DATA_BLOCK "Segnal Avvisi Allarmi OP"
TITLE =Segnalazioni Avvisi Allarmi OP17
AUTHOR : MassimoZ
FAMILY : NovaSrl
VERSION : 0.1


  STRUCT
   Avviso : BOOL ;	//Manca Marcia Generale
   Avviso1 : BOOL ;	//Barriere di sicurezza aperte
   Avviso2 : BOOL ;	//Protezioni anteriori aperte
   Avviso3 : BOOL ;	//Blocco cancello attivo
   Avviso4 : BOOL ;	//spare
   Avviso5 : BOOL ;	//spare
   Avviso6 : BOOL ;	//spare
   Avviso7 : BOOL ;	//spare
   Avviso8 : BOOL ;	//spare
   Avviso9 : BOOL ;	//spare
   Avviso10 : BOOL ;	//spare
   Avviso11 : BOOL ;	//spare
   Avviso12 : BOOL ;	//spare
   Avviso13 : BOOL ;	//spare
   Avviso14 : BOOL ;	//spare
   Avviso15 : BOOL ;	//spare
   Avviso16 : BOOL ;	//Inserito Arresto a Fine Ciclo
   Avviso17 : BOOL ;	//Eseguire Ref Point Assi
   Avviso18 : BOOL ;	//Testa Fuori Posizione Base per il Ciclo Aut
   Avviso19 : BOOL ;	//Testa Fuori Posizione Base per il Ciclo S/Aut
   Avviso20 : BOOL ;	//spare
   Avviso21 : BOOL ;	//spare
   Avviso22 : BOOL ;	//spare
   Avviso23 : BOOL ;	//Controllo corti escluso Escluso
   Avviso24 : BOOL ;	//Macchin in ingombro
   Avviso25 : BOOL ;	//Batteria Tampone Plc Scarica
   Avviso26 : BOOL ;
   Avviso27 : BOOL ;
   Avviso28 : BOOL ;
   Avviso29 : BOOL ;
   Avviso30 : BOOL ;
   Avviso31 : BOOL ;
   Avviso32 : BOOL ;
   Avviso33 : BOOL ;
   Avviso34 : BOOL ;
   Avviso35 : BOOL ;
   Avviso36 : BOOL ;
   Avviso37 : BOOL ;
   Avviso38 : BOOL ;
   Avviso39 : BOOL ;
   Avviso40 : BOOL ;
   Avviso41 : BOOL ;
   Avviso42 : BOOL ;
   Avviso43 : BOOL ;
   Avviso44 : BOOL ;
   Avviso45 : BOOL ;
   Avviso46 : BOOL ;
   Avviso47 : BOOL ;
   Avviso48 : BOOL ;
   Avviso49 : BOOL ;
   Avviso50 : BOOL ;
   Avviso51 : BOOL ;
   Avviso52 : BOOL ;
   Avviso53 : BOOL ;
   Avviso54 : BOOL ;
   Avviso55 : BOOL ;
   Avviso56 : BOOL ;
   Avviso57 : BOOL ;
   Avviso58 : BOOL ;
   Avviso59 : BOOL ;
   Avviso60 : BOOL ;
   Avviso61 : BOOL ;
   Avviso62 : BOOL ;
   Avviso63 : BOOL ;
   Allarme : BOOL ;	//Alimentazione Ausiliari 110Vac
   Allarme1 : BOOL ;	//Scatto termico IM1
   Allarme2 : BOOL ;	//Scatto termico IM2
   Allarme3 : BOOL ;	//Scatto termico IM3
   Allarme4 : BOOL ;	//Mancato ritorno TL4
   Allarme5 : BOOL ;	//Scatto termico IM4
   Allarme6 : BOOL ;	//Spare
   Allarme7 : BOOL ;	//Spare
   Allarme8 : BOOL ;	//Spare
   Allarme9 : BOOL ;	//Spare
   Allarme10 : BOOL ;	//Spare
   Allarme11 : BOOL ;	//Spare
   Allarme12 : BOOL ;	//Spare
   Allarme13 : BOOL ;	//Spare
   Allarme14 : BOOL ;	//Spare
   Allarme15 : BOOL ;	//Spare
   Allarme16 : BOOL ;	//Spare
   Allarme17 : BOOL ;	//Spare
   Allarme18 : BOOL ;	//Spare
   Allarme19 : BOOL ;	//Spare
   Allarme20 : BOOL ;	//Spare
   Allarme21 : BOOL ;	//Spare
   Allarme22 : BOOL ;	//Spare
   Allarme23 : BOOL ;	//Spare
   Allarme24 : BOOL ;	//Spare
   Allarme25 : BOOL ;	//Spare
   Allarme26 : BOOL ;	//Spare
   Allarme27 : BOOL ;	//Spare
   Allarme28 : BOOL ;	//Spare
   Allarme29 : BOOL ;	//Spare
   Allarme30 : BOOL ;	//Spare
   Allarme31 : BOOL ;	//Spare
   Allarme32 : BOOL ;	//Spare
   Allarme33 : BOOL ;	//Spare
   Allarme34 : BOOL ;	//Spare
   Allarme35 : BOOL ;	//Spare
   Allarme36 : BOOL ;	//Spare
   Allarme37 : BOOL ;	//Spare
   Allarme38 : BOOL ;	//Spare
   Allarme39 : BOOL ;	//Spare
   Allarme40 : BOOL ;	//Spare
   Allarme41 : BOOL ;	//Spare
   Allarme42 : BOOL ;	//Spare
   Allarme43 : BOOL ;	//Spare
   Allarme44 : BOOL ;	//Spare
   Allarme45 : BOOL ;	//Spare
   Allarme46 : BOOL ;	//Spare
   Allarme47 : BOOL ;	//Spare
   Allarme48 : BOOL ;	//Spare
   Allarme49 : BOOL ;	//Spare
   Allarme50 : BOOL ;	//Spare
   Allarme51 : BOOL ;
   Allarme52 : BOOL ;
   Allarme53 : BOOL ;
   Allarme54 : BOOL ;
   Allarme55 : BOOL ;
   Allarme56 : BOOL ;
   Allarme57 : BOOL ;
   Allarme58 : BOOL ;
   Allarme59 : BOOL ;
   Allarme60 : BOOL ;
   Allarme61 : BOOL ;
   Allarme62 : BOOL ;
   Allarme63 : BOOL ;
   Allarme64 : BOOL ;
   Allarme65 : BOOL ;
   Allarme66 : BOOL ;
   Allarme67 : BOOL ;
   Allarme68 : BOOL ;
   Allarme69 : BOOL ;
   Allarme70 : BOOL ;
   Allarme71 : BOOL ;
   Allarme72 : BOOL ;
   Allarme73 : BOOL ;
   Allarme74 : BOOL ;
   Allarme75 : BOOL ;
   Allarme76 : BOOL ;
   Allarme77 : BOOL ;
   Allarme78 : BOOL ;
   Allarme79 : BOOL ;
   Allarme80 : BOOL ;
   Allarme81 : BOOL ;
   Allarme82 : BOOL ;
   Allarme83 : BOOL ;
   Allarme84 : BOOL ;
   Allarme85 : BOOL ;
   Allarme86 : BOOL ;
   Allarme87 : BOOL ;
   Allarme88 : BOOL ;
   Allarme89 : BOOL ;
   Allarme90 : BOOL ;
   Allarme91 : BOOL ;
   Allarme92 : BOOL ;
   Allarme93 : BOOL ;
   Allarme94 : BOOL ;
   Allarme95 : BOOL ;
   AcquPlc : WORD ;	//Acquisizione Allarmi Plc
   AcquPlc1 : WORD ;	//Acquisizione Allarmi Plc
   AcquPlc2 : WORD ;	//Acquisizione Allarmi Plc
   AcquPlc3 : WORD ;	//Acquisizione Allarmi Plc
   AcquPlc4 : WORD ;	//Acquisizione Allarmi Plc
   AcquPlc5 : WORD ;	//Acquisizione Allarmi Plc
  END_STRUCT ;
BEGIN
   Avviso := FALSE;
   Avviso1 := FALSE;
   Avviso2 := FALSE;
   Avviso3 := FALSE;
   Avviso4 := FALSE;
   Avviso5 := FALSE;
   Avviso6 := FALSE;
   Avviso7 := FALSE;
   Avviso8 := FALSE;
   Avviso9 := FALSE;
   Avviso10 := FALSE;
   Avviso11 := FALSE;
   Avviso12 := FALSE;
   Avviso13 := FALSE;
   Avviso14 := FALSE;
   Avviso15 := FALSE;
   Avviso16 := FALSE;
   Avviso17 := FALSE;
   Avviso18 := FALSE;
   Avviso19 := FALSE;
   Avviso20 := FALSE;
   Avviso21 := FALSE;
   Avviso22 := FALSE;
   Avviso23 := FALSE;
   Avviso24 := FALSE;
   Avviso25 := FALSE;
   Avviso26 := FALSE;
   Avviso27 := FALSE;
   Avviso28 := FALSE;
   Avviso29 := FALSE;
   Avviso30 := FALSE;
   Avviso31 := FALSE;
   Avviso32 := FALSE;
   Avviso33 := FALSE;
   Avviso34 := FALSE;
   Avviso35 := FALSE;
   Avviso36 := FALSE;
   Avviso37 := FALSE;
   Avviso38 := FALSE;
   Avviso39 := FALSE;
   Avviso40 := FALSE;
   Avviso41 := FALSE;
   Avviso42 := FALSE;
   Avviso43 := FALSE;
   Avviso44 := FALSE;
   Avviso45 := FALSE;
   Avviso46 := FALSE;
   Avviso47 := FALSE;
   Avviso48 := FALSE;
   Avviso49 := FALSE;
   Avviso50 := FALSE;
   Avviso51 := FALSE;
   Avviso52 := FALSE;
   Avviso53 := FALSE;
   Avviso54 := FALSE;
   Avviso55 := FALSE;
   Avviso56 := FALSE;
   Avviso57 := FALSE;
   Avviso58 := FALSE;
   Avviso59 := FALSE;
   Avviso60 := FALSE;
   Avviso61 := FALSE;
   Avviso62 := FALSE;
   Avviso63 := FALSE;
   Allarme := FALSE;
   Allarme1 := FALSE;
   Allarme2 := FALSE;
   Allarme3 := FALSE;
   Allarme4 := FALSE;
   Allarme5 := FALSE;
   Allarme6 := FALSE;
   Allarme7 := FALSE;
   Allarme8 := FALSE;
   Allarme9 := FALSE;
   Allarme10 := FALSE;
   Allarme11 := FALSE;
   Allarme12 := FALSE;
   Allarme13 := FALSE;
   Allarme14 := FALSE;
   Allarme15 := FALSE;
   Allarme16 := FALSE;
   Allarme17 := FALSE;
   Allarme18 := FALSE;
   Allarme19 := FALSE;
   Allarme20 := FALSE;
   Allarme21 := FALSE;
   Allarme22 := FALSE;
   Allarme23 := FALSE;
   Allarme24 := FALSE;
   Allarme25 := FALSE;
   Allarme26 := FALSE;
   Allarme27 := FALSE;
   Allarme28 := FALSE;
   Allarme29 := FALSE;
   Allarme30 := FALSE;
   Allarme31 := FALSE;
   Allarme32 := FALSE;
   Allarme33 := FALSE;
   Allarme34 := FALSE;
   Allarme35 := FALSE;
   Allarme36 := FALSE;
   Allarme37 := FALSE;
   Allarme38 := FALSE;
   Allarme39 := FALSE;
   Allarme40 := FALSE;
   Allarme41 := FALSE;
   Allarme42 := FALSE;
   Allarme43 := FALSE;
   Allarme44 := FALSE;
   Allarme45 := FALSE;
   Allarme46 := FALSE;
   Allarme47 := FALSE;
   Allarme48 := FALSE;
   Allarme49 := FALSE;
   Allarme50 := FALSE;
   Allarme51 := FALSE;
   Allarme52 := FALSE;
   Allarme53 := FALSE;
   Allarme54 := FALSE;
   Allarme55 := FALSE;
   Allarme56 := FALSE;
   Allarme57 := FALSE;
   Allarme58 := FALSE;
   Allarme59 := FALSE;
   Allarme60 := FALSE;
   Allarme61 := FALSE;
   Allarme62 := FALSE;
   Allarme63 := FALSE;
   Allarme64 := FALSE;
   Allarme65 := FALSE;
   Allarme66 := FALSE;
   Allarme67 := FALSE;
   Allarme68 := FALSE;
   Allarme69 := FALSE;
   Allarme70 := FALSE;
   Allarme71 := FALSE;
   Allarme72 := FALSE;
   Allarme73 := FALSE;
   Allarme74 := FALSE;
   Allarme75 := FALSE;
   Allarme76 := FALSE;
   Allarme77 := FALSE;
   Allarme78 := FALSE;
   Allarme79 := FALSE;
   Allarme80 := FALSE;
   Allarme81 := FALSE;
   Allarme82 := FALSE;
   Allarme83 := FALSE;
   Allarme84 := FALSE;
   Allarme85 := FALSE;
   Allarme86 := FALSE;
   Allarme87 := FALSE;
   Allarme88 := FALSE;
   Allarme89 := FALSE;
   Allarme90 := FALSE;
   Allarme91 := FALSE;
   Allarme92 := FALSE;
   Allarme93 := FALSE;
   Allarme94 := FALSE;
   Allarme95 := FALSE;
   AcquPlc := W#16#FFFF;
   AcquPlc1 := W#16#FFFF;
   AcquPlc2 := W#16#FFFF;
   AcquPlc3 := W#16#FFFF;
   AcquPlc4 := W#16#FFFF;
   AcquPlc5 := W#16#FFFF;
END_DATA_BLOCK

